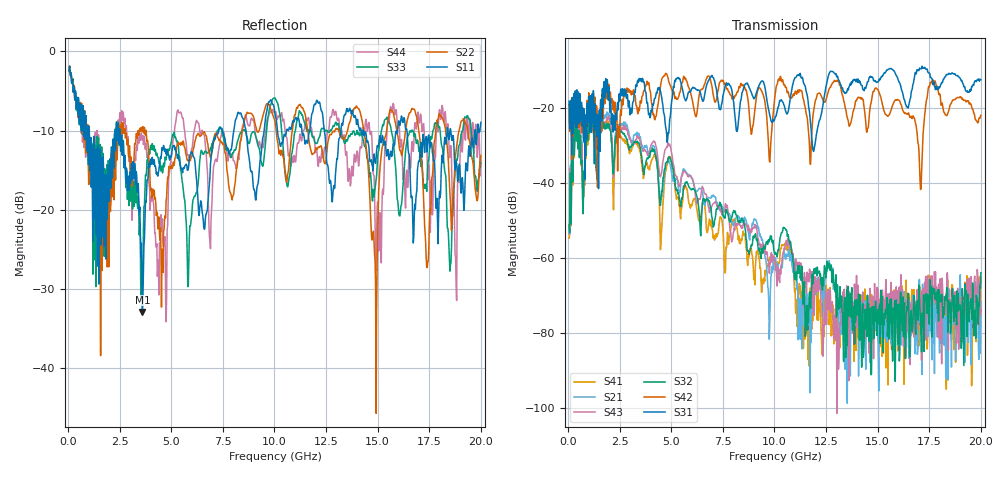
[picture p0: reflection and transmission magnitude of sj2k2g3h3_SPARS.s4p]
! FILE: E:\users\goganessyan\GBX_Backplane\FR408_backplane\1m_OUTBOUND_FEXT\sj2k2g3h3_SPARS.s4p
# MHZ S RI R 50.00
! FREQ  S11  S12  S13  S14
!  S21  S22  S23  S24
!  S31  S32  S33  S34
!  S41  S42  S43  S44
!  REAL  IMAG  REAL  IMAG  REAL  IMAG  REAL  IMAG
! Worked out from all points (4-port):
!   799 points, 50 MHz to 20 GHz, reference 50 ohm
!   strongest paths, dB at 50 MHz, 5.025 GHz, 10.03 GHz, 15.03 GHz, 20 GHz:
!     S31: -18.3, -18.0, -22.7, -13.1, -12.6
!     S42: -19.2, -15.1, -16.8, -15.4, -22.0
!     S32: -51.2, -34.7, -59.0, -77.6, -63.9
!     S43: -53.5, -32.4, -60.8, -68.3, -73.8
!     S21: -51.7, -37.6, -59.9, -84.7, -71.6
!     S41: -54.7, -35.0, -62.0, -81.4, -75.4
!   lowest |S11| = -32.9 dB at 3.6 GHz (marker M1), VSWR 1.05, Z = 50.4 + j2.24 ohm
!   |S11| at or under -10 dB: 2.506 GHz to 7.303 GHz (4.796 GHz wide, 97.8 % of centre); 14.3 GHz to 15.96 GHz (1.661 GHz wide, 11 % of centre); 16.42 GHz to 18.37 GHz (1.951 GHz wide, 11.2 % of centre)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
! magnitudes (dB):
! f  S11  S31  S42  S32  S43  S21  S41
! 50 MHz  -2.5  -18.3  -19.2  -51.2  -53.5  -51.7  -54.7
! 425 MHz  -5.8  -15.3  -16.4  -24.9  -23.4  -22.9  -25.3
! 3.6 GHz  -32.9  -12.2  -16.9  -34.7  -31.2  -30.3  -36.5
! 11.18 GHz  -8.5  -11.3  -16.0  -64.1  -61.9  -77.5  -69.5
! 14.9 GHz  -14.1  -12.9  -14.8  -71.5  -74.8  -71.6  -72.5
! 15.62 GHz  -12.6  -9.6  -21.1  -77.0  -69.2  -74.7  -69.6
! 20 GHz  -9.0  -12.6  -22.0  -63.9  -73.8  -71.6  -75.4
